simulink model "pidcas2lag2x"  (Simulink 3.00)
settings: Solver=ode45  SolverMode=SingleTasking  StartTime=0.0  StopTime=100  FixedStep=st_size  MaxStep=st_size  RelTol=1e-5  AbsTol=1e-6
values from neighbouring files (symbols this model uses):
  Disturb = Setpoint    [mimo_MSF1DF_sim.m]    (also in mimo_MSF2DF_sim.m)
  Satlb = temp1    [cback.m]    (also in imcmenu.m = str2num(satlbs))
  Satub = temp1    [cback.m]    (also in imcmenu.m = str2num(satubs))
  Setpoint = zeros(1,n)    [mimo_MSF1DF_sim.m]    (also in mimo_MSF2DF_sim.m)
undefined symbols (not defined in the file or in its folder): a1, a2, b1, b2, conv, denCs2, K1, keps, numCs2, Qdden, TauD1, TauI1, XdenPs, XnumPs, Xpdeadx

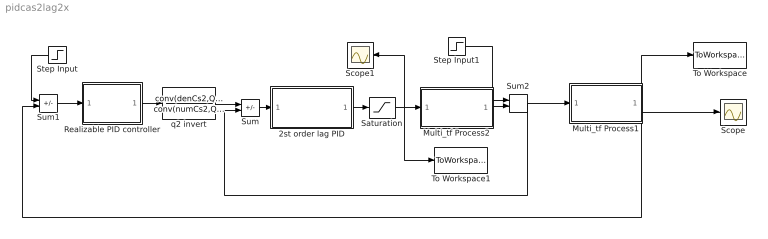
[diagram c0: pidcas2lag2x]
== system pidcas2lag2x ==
  2st order lag PID : Subsystem
  Multi_tf Process1 : Subsystem
  Multi_tf Process2 : Subsystem
  Realizable PID controller : Subsystem
  Saturation : Saturate  UpperLimit=Satub  LowerLimit=Satlb
  Scope : Scope
  Scope1 : Scope
  Step Input : Step  Orientation=left  Time=0  Before=0  After=Setpoint  SampleTime=0
  Step Input1 : Step  Time=0  Before=0  After=Disturb  SampleTime=0
  Sum : Sum  Inputs=+-  SaturateOnIntegerOverflow=on
  Sum1 : Sum  Inputs=+-  SaturateOnIntegerOverflow=on
  Sum2 : Sum  Inputs=++  SaturateOnIntegerOverflow=on
  To Workspace : ToWorkspace  VariableName=simout  SampleTime=-1  SaveFormat=Matrix
  To Workspace1 : ToWorkspace  VariableName=effort  SampleTime=-1  SaveFormat=Matrix
  q2 invert : TransferFcn  Numerator=conv(denCs2,Qdden)  Denominator=conv(numCs2,Qdden)
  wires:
  Sum/1 -> 2st order lag PID/1(In1)
  Multi_tf Process2/1(Out1) -> Sum2/2
  Step Input1/1 -> Sum2/1
  2st order lag PID/1(Out1) -> Saturation/1
  Saturation/1 -> To Workspace1/1, Multi_tf Process2/1(In1), Scope1/1
  Sum2/1 -> Sum/2, Multi_tf Process1/1(In1)
  Step Input/1 -> Sum1/1
  Sum1/1 -> Realizable PID controller/1(In1)
  q2 invert/1 -> Sum/1
  Realizable PID controller/1(Out1) -> q2 invert/1
  Multi_tf Process1/1(Out1) -> Sum1/2, To Workspace/1, Scope/1

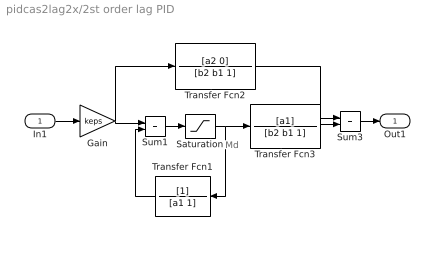
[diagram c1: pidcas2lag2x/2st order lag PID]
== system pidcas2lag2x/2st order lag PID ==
  note: Md
  In1 : Inport  Port=1  PortWidth=-1  SampleTime=-1  DataType=auto
  Gain : Gain  Gain=keps  SaturateOnIntegerOverflow=on
  Saturation : Saturate  UpperLimit=Satub  LowerLimit=Satlb
  Sum1 : Sum  Inputs=++  SaturateOnIntegerOverflow=on
  Sum3 : Sum  Inputs=++  SaturateOnIntegerOverflow=on
  Transfer Fcn1 : TransferFcn  Orientation=left  Numerator=[1]  Denominator=[a1 1]
  Transfer Fcn2 : TransferFcn  Numerator=[a2 0]  Denominator=[b2 b1 1]
  Transfer Fcn3 : TransferFcn  Numerator=[a1]  Denominator=[b2 b1 1]
  Out1 : Outport  Port=1  InitialOutput=0
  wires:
  Gain/1 -> Transfer Fcn2/1, Sum1/1
  Transfer Fcn1/1 -> Sum1/2
  Saturation/1 -> Transfer Fcn1/1, Transfer Fcn3/1
  Sum1/1 -> Saturation/1
  Transfer Fcn3/1 -> Sum3/2
  In1/1 -> Gain/1
  Sum3/1 -> Out1/1
  Transfer Fcn2/1 -> Sum3/1

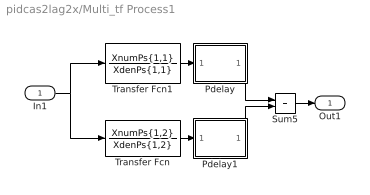
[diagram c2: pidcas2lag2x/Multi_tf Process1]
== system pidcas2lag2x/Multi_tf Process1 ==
  In1 : Inport  Port=1  PortWidth=-1  SampleTime=-1  DataType=auto
  Pdelay : Subsystem
  Pdelay1 : Subsystem
  Sum5 : Sum  Inputs=++  SaturateOnIntegerOverflow=on
  Transfer Fcn : TransferFcn  Numerator=XnumPs{1,2}  Denominator=XdenPs{1,2}
  Transfer Fcn1 : TransferFcn  Numerator=XnumPs{1,1}  Denominator=XdenPs{1,1}
  Out1 : Outport  Port=1  InitialOutput=0
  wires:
  Transfer Fcn1/1 -> Pdelay/1(In1)
  Transfer Fcn/1 -> Pdelay1/1(In1)
  Pdelay/1(Out1) -> Sum5/1
  In1/1 -> Transfer Fcn1/1, Transfer Fcn/1
  Sum5/1 -> Out1/1
  Pdelay1/1(Out1) -> Sum5/2

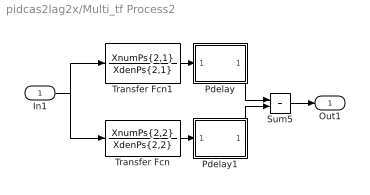
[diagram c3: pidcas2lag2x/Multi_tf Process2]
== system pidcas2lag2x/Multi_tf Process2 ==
  In1 : Inport  Port=1  PortWidth=-1  SampleTime=-1  DataType=auto
  Pdelay : Subsystem
  Pdelay1 : Subsystem
  Sum5 : Sum  Inputs=++  SaturateOnIntegerOverflow=on
  Transfer Fcn : TransferFcn  Numerator=XnumPs{2,2}  Denominator=XdenPs{2,2}
  Transfer Fcn1 : TransferFcn  Numerator=XnumPs{2,1}  Denominator=XdenPs{2,1}
  Out1 : Outport  Port=1  InitialOutput=0
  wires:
  Transfer Fcn1/1 -> Pdelay/1(In1)
  Transfer Fcn/1 -> Pdelay1/1(In1)
  Pdelay/1(Out1) -> Sum5/1
  Pdelay1/1(Out1) -> Sum5/2
  In1/1 -> Transfer Fcn1/1, Transfer Fcn/1
  Sum5/1 -> Out1/1

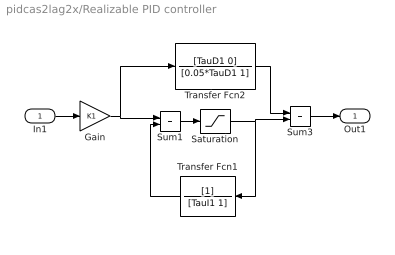
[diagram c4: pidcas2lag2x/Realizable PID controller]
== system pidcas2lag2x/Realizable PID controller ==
  In1 : Inport  Port=1  PortWidth=-1  SampleTime=-1  DataType=auto
  Gain : Gain  Gain=K1  SaturateOnIntegerOverflow=on
  Saturation : Saturate  UpperLimit=Satub  LowerLimit=Satlb
  Sum1 : Sum  Inputs=++  SaturateOnIntegerOverflow=on
  Sum3 : Sum  Inputs=++  SaturateOnIntegerOverflow=on
  Transfer Fcn1 : TransferFcn  Orientation=left  Numerator=[1]  Denominator=[TauI1 1]
  Transfer Fcn2 : TransferFcn  Numerator=[TauD1 0]  Denominator=[0.05*TauD1 1]
  Out1 : Outport  Port=1  InitialOutput=0
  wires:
  Transfer Fcn1/1 -> Sum1/2
  Transfer Fcn2/1 -> Sum3/1
  Sum3/1 -> Out1/1
  In1/1 -> Gain/1
  Gain/1 -> Sum1/1, Transfer Fcn2/1
  Sum1/1 -> Saturation/1
  Saturation/1 -> Sum3/2, Transfer Fcn1/1

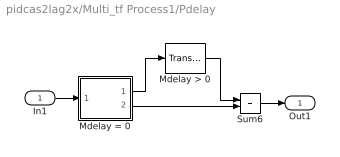
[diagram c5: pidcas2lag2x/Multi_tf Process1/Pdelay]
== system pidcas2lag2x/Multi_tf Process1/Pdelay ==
  In1 : Inport  Port=1  PortWidth=-1  SampleTime=-1  DataType=auto
  Mdelay > 0 : TransportDelay  DelayTime=Xpdeadx{1,1}  InitialInput=0  BufferSize=1024
  Mdelay = 0 : Subsystem  Description=pass input signal through out1 if condition is true.
  Sum6 : Sum  Inputs=++  SaturateOnIntegerOverflow=on
  Out1 : Outport  Port=1
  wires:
  Mdelay = 0/1(Out2) -> Mdelay > 0/1
  Mdelay > 0/1 -> Sum6/1
  Mdelay = 0/2(Out1) -> Sum6/2
  In1/1 -> Mdelay = 0/1(In)
  Sum6/1 -> Out1/1

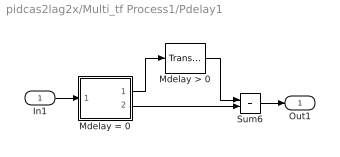
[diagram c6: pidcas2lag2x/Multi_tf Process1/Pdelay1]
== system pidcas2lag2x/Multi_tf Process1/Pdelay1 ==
  In1 : Inport  Port=1  PortWidth=-1  SampleTime=-1  DataType=auto
  Mdelay > 0 : TransportDelay  DelayTime=Xpdeadx{1,2}  InitialInput=0  BufferSize=1024
  Mdelay = 0 : Subsystem  Description=pass input signal through out1 if condition is true.
  Sum6 : Sum  Inputs=++  SaturateOnIntegerOverflow=on
  Out1 : Outport  Port=1
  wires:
  Mdelay = 0/1(Out2) -> Mdelay > 0/1
  Mdelay > 0/1 -> Sum6/1
  Mdelay = 0/2(Out1) -> Sum6/2
  In1/1 -> Mdelay = 0/1(In)
  Sum6/1 -> Out1/1

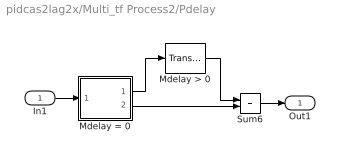
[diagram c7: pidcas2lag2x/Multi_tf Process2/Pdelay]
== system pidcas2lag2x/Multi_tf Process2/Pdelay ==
  In1 : Inport  Port=1  PortWidth=-1  SampleTime=-1  DataType=auto
  Mdelay > 0 : TransportDelay  DelayTime=Xpdeadx{2,1}  InitialInput=0  BufferSize=1024
  Mdelay = 0 : Subsystem  Description=pass input signal through out1 if condition is true.
  Sum6 : Sum  Inputs=++  SaturateOnIntegerOverflow=on
  Out1 : Outport  Port=1
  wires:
  Mdelay = 0/1(Out2) -> Mdelay > 0/1
  Mdelay > 0/1 -> Sum6/1
  Mdelay = 0/2(Out1) -> Sum6/2
  In1/1 -> Mdelay = 0/1(In)
  Sum6/1 -> Out1/1

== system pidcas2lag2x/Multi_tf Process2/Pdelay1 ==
  In1 : Inport  Port=1  PortWidth=-1  SampleTime=-1  DataType=auto
  Mdelay > 0 : TransportDelay  DelayTime=Xpdeadx{2,2}  InitialInput=0  BufferSize=1024
  Mdelay = 0 : Subsystem  Description=pass input signal through out1 if condition is true.
  Sum6 : Sum  Inputs=++  SaturateOnIntegerOverflow=on
  Out1 : Outport  Port=1
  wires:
  Mdelay = 0/1(Out2) -> Mdelay > 0/1
  Mdelay > 0/1 -> Sum6/1
  Mdelay = 0/2(Out1) -> Sum6/2
  In1/1 -> Mdelay = 0/1(In)
  Sum6/1 -> Out1/1

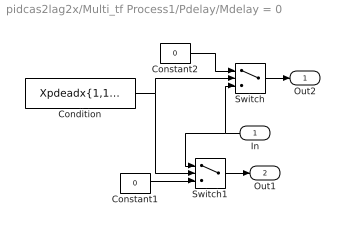
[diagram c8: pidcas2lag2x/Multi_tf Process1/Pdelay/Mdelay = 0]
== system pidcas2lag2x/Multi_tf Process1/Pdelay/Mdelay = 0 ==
  In : Inport  Orientation=left  Port=1  PortWidth=-1  SampleTime=-1  DataType=auto
  Condition : Constant  Value=Xpdeadx{1,1}<=3*eps
  Constant1 : Constant  Value=0
  Constant2 : Constant  Value=0
  Switch : Switch  Threshold=1
  Switch1 : Switch  Threshold=1
  Out2 : Outport  Port=1  InitialOutput=0
  Out1 : Outport  Port=2  InitialOutput=0
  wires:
  In/1 -> Switch/3, Switch1/1
  Condition/1 -> Switch1/2, Switch/2
  Constant1/1 -> Switch1/3
  Constant2/1 -> Switch/1
  Switch/1 -> Out2/1
  Switch1/1 -> Out1/1

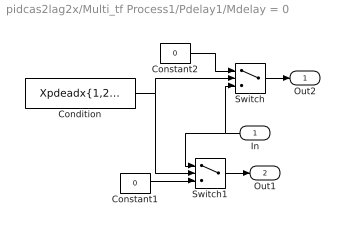
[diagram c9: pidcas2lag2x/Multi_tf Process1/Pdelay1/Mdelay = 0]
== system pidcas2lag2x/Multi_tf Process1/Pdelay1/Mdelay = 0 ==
  In : Inport  Orientation=left  Port=1  PortWidth=-1  SampleTime=-1  DataType=auto
  Condition : Constant  Value=Xpdeadx{1,2}<=3*eps
  Constant1 : Constant  Value=0
  Constant2 : Constant  Value=0
  Switch : Switch  Threshold=1
  Switch1 : Switch  Threshold=1
  Out2 : Outport  Port=1  InitialOutput=0
  Out1 : Outport  Port=2  InitialOutput=0
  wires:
  In/1 -> Switch/3, Switch1/1
  Condition/1 -> Switch1/2, Switch/2
  Constant1/1 -> Switch1/3
  Constant2/1 -> Switch/1
  Switch/1 -> Out2/1
  Switch1/1 -> Out1/1

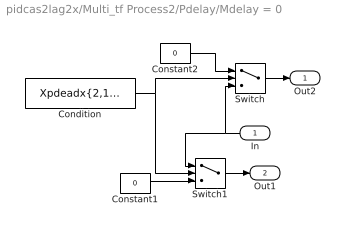
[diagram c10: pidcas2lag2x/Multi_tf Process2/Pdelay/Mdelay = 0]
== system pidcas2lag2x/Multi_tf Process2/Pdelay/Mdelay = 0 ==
  In : Inport  Orientation=left  Port=1  PortWidth=-1  SampleTime=-1  DataType=auto
  Condition : Constant  Value=Xpdeadx{2,1}<=3*eps
  Constant1 : Constant  Value=0
  Constant2 : Constant  Value=0
  Switch : Switch  Threshold=1
  Switch1 : Switch  Threshold=1
  Out2 : Outport  Port=1  InitialOutput=0
  Out1 : Outport  Port=2  InitialOutput=0
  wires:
  In/1 -> Switch/3, Switch1/1
  Condition/1 -> Switch1/2, Switch/2
  Constant1/1 -> Switch1/3
  Constant2/1 -> Switch/1
  Switch/1 -> Out2/1
  Switch1/1 -> Out1/1

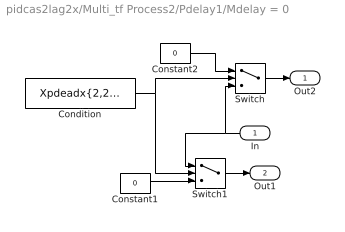
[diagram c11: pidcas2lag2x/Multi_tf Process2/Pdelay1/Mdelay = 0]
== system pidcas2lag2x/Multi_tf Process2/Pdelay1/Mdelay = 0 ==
  In : Inport  Orientation=left  Port=1  PortWidth=-1  SampleTime=-1  DataType=auto
  Condition : Constant  Value=Xpdeadx{2,2}<=3*eps
  Constant1 : Constant  Value=0
  Constant2 : Constant  Value=0
  Switch : Switch  Threshold=1
  Switch1 : Switch  Threshold=1
  Out2 : Outport  Port=1  InitialOutput=0
  Out1 : Outport  Port=2  InitialOutput=0
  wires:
  In/1 -> Switch/3, Switch1/1
  Condition/1 -> Switch1/2, Switch/2
  Constant1/1 -> Switch1/3
  Constant2/1 -> Switch/1
  Switch/1 -> Out2/1
  Switch1/1 -> Out1/1
